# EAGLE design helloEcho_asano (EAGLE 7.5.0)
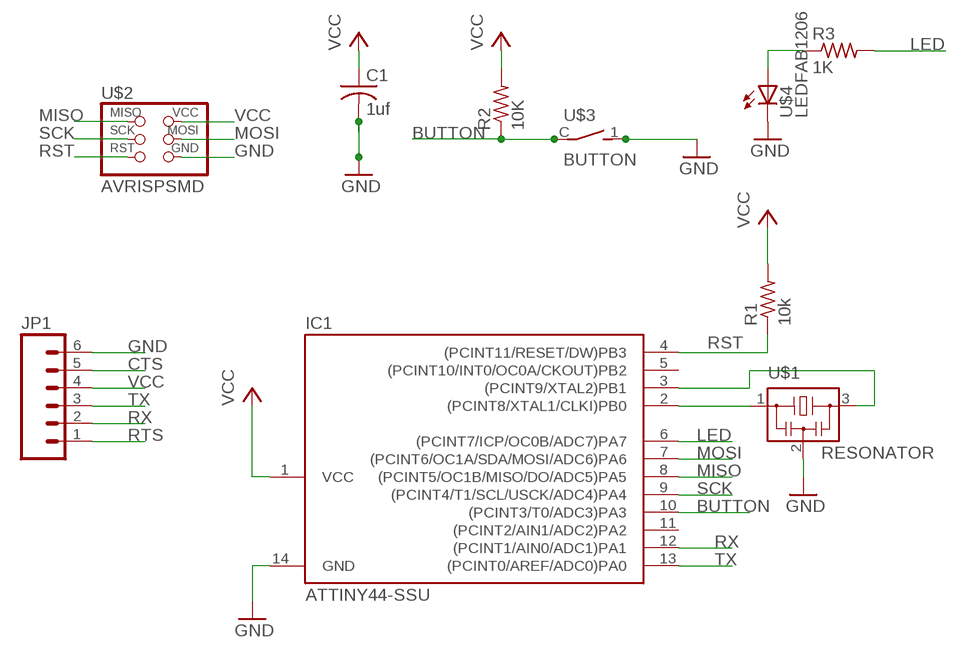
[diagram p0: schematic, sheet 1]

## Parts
C1  1uf  C-USC1206  [C1206]
IC1  ATTINY44-SSU  [SOIC14]
JP1  M06SMD  [1X06-SMD]
R1  10k  R-US_R1206  [R1206]
R2  10K  RES-US1206FAB  [R1206FAB]
R3  1K  RES-US1206FAB  [R1206FAB]
U$1  RESONATOR  [EFOBM]
U$2  AVRISPSMD  [2X03SMD]
U$3  BUTTON  [BUT-NPS]
U$4  LEDFAB1206  [LED1206FAB]

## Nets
BUTTON: IC1.10((PCINT3/T0/ADC3)PA3) R2.1 U$3.C
CTS: JP1.5
GND: C1.2 IC1.14(GND) JP1.6 U$1.2 U$2.6(GND) U$3.1 U$4.2(C)
LED: IC1.6((PCINT7/ICP/OC0B/ADC7)PA7) R3.2
MISO: IC1.8((PCINT5/OC1B/MISO/DO/ADC5)PA5) U$2.1(MISO)
MOSI: IC1.7((PCINT6/OC1A/SDA/MOSI/ADC6)PA6) U$2.4(MOSI)
N$1: IC1.2((PCINT8/XTAL1/CLKI)PB0) U$1.1
N$2: IC1.3((PCINT9/XTAL2)PB1) U$1.3
N$3: R3.1 U$4.1(A)
RST: IC1.4((PCINT11/RESET/DW)PB3) R1.1 U$2.5(RST)
RTS: JP1.1
RX: IC1.12((PCINT1/AIN0/ADC1)PA1) JP1.2
SCK: IC1.9((PCINT4/T1/SCL/USCK/ADC4)PA4) U$2.3(SCK)
TX: IC1.13((PCINT0/AREF/ADC0)PA0) JP1.3
VCC: C1.1 IC1.1(VCC) JP1.4 R1.2 R2.2 U$2.2(VCC)
Unconnected: IC1.5((PCINT10/INT0/OC0A/CKOUT)PB2) IC1.11((PCINT2/AIN1/ADC2)PA2)

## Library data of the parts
C1 = rcl:C-US: CAPACITOR, American symbol
IC1 = fab:ATTINY44
JP1 = SparkFun:M06: Header 6 Standard 6-pin 0.1" header. Use with straight break away headers (SKU : PRT-00116), right angle break away headers (PRT-00553), swiss pins (PRT-00743), machine pins (PRT-00117), and female headers (PRT-00115). Molex polarized connector foot print use with SKU : PRT-08094 with associated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
R1 = resistor:R-US_: RESISTOR, American symbol
R2 R3 = HelloKamakura:RES-US: Resistor (US Symbol)
U$1 = fab:RESONATOR
U$2 = fab:AVRISP
U$3 = HelloKamakura:BUTTON: Distribute : Akizuki Densi
U$4 = HelloKamakura:LED: LED

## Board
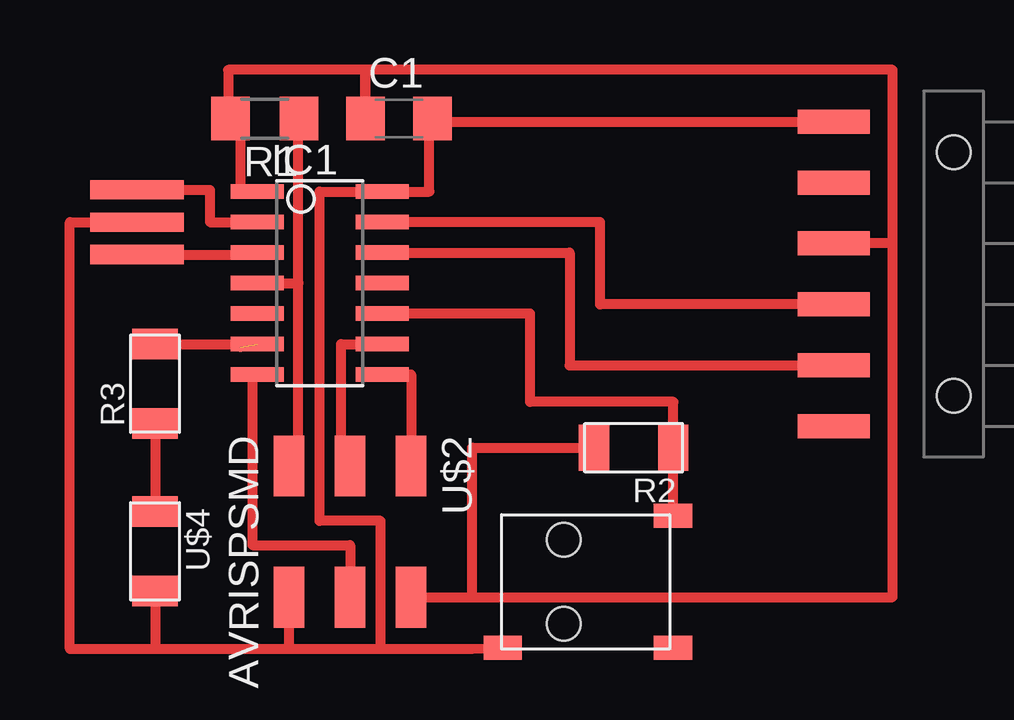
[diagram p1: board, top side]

No outline drawn. Coordinates in mm, seen from the top.
Copper layers 1: Top 0.035mm
Design rules "ERP-1sided-10mil-16mill": minimum track width 10mil, minimum drill 24mil, track to track 16mil, track to pad 16mil, pad to pad 16mil, via to via 16mil, smd to smd 0mil, copper to edge 16mil, drill to drill 36mil, minimum pad ring 10mil, minimum via ring 8mil, stop-mask expansion 4mil, vias tented up to drill 0mil, thermal gap 10mil

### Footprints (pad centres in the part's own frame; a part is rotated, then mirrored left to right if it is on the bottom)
C1206 = smd 1.6 x 1.8: 1 -1.4,0; 2 1.4,0
SOIC14 = smd 0.61 x 2.21: 1 -3.81,-2.603; 2 -2.54,-2.603; 3 -1.27,-2.603; 4 0,-2.603; 5 1.27,-2.603; 6 2.54,-2.603; 7 3.81,-2.603; 8 3.81,2.603; 9 2.54,2.603; 10 1.27,2.603; 11 0,2.603; 12 -1.27,2.603; 13 -2.54,2.603; 14 -3.81,2.603
1X06-SMD = smd 1 x 3: 1 -6.35,5; 2 -3.81,5; 3 -1.27,5; 4 1.27,5; 5 3.81,5; 6 6.35,5 | hole 1.4: -5.08,0; 5.08,0
R1206 = smd 1.6 x 1.803: 1 -1.422,0; 2 1.422,0
R1206FAB = smd 1.27 x 1.905: 1 -1.651,0; 2 1.651,0
EFOBM = smd 0.8 x 3.9: 1 -1.35,0; 2 0,0; 3 1.35,0
2X03SMD = smd 2.54 x 1.27: 1 -2.54,2.54; 2 2.92,2.54; 3 -2.54,0; 4 2.92,0; 5 -2.54,-2.54; 6 2.92,-2.54
BUT-NPS = smd 1 x 1.6: 1 2.75,-3.55; C -2.75,3.55; P$1 2.75,3.55 | hole 1.4: -1.75,-1; 1.75,-1
LED1206FAB = smd 1.27 x 1.905: 1 -1.651,0; 2 1.651,0

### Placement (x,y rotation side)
C1  29.72,40.51 0 top
IC1  26.42,33.66 270 top
JP1  52.83,34.04 90 top
R1  24.13,40.51 180 top
R2  39.5,26.8 180 top
R3  19.56,29.46 90 top
U$1  18.8,36.2 270 top
U$2  27.69,23.5 270 top
U$3  37.59,21.21 270 top
U$4  19.56,22.48 270 top

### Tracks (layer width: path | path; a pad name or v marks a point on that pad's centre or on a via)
BUTTON
  Top 0.406: U$3.C R2.1 41.15,28.7 35.18,28.7 35.18,32.38 IC1.10
GND
  Top 0.406: 28.96,18.41 28.96,23.75 26.42,23.75 26.42,37.47 IC1.14 30.99,37.47 30.99,40.51 C1.2 31.12,40.39 JP1.6 47.83,40.64 | 25.15,18.41 28.96,18.41 | U$1.2 16,36.2 16,18.41 19.56,18.41 | U$2.6 25.15,18.41 | 19.56,18.41 25.15,18.41 | 28.96,18.41 32.77,18.41 U$3.1 | U$4.2 19.56,18.41
LED  (1 unrouted)
  Top 0.406: R3.2 23.11,31.11 23.11,30.99
MISO
  Top 0.406: IC1.8 30.23,29.84 U$2.1
MOSI
  Top 0.406: IC1.7 23.62,29.84 23.62,22.73 27.69,22.73 U$2.4
N$1
  Top 0.406: U$1.1 21.84,37.55 21.84,36.2 IC1.2
N$2
  Top 0.406: U$1.3 23.81,34.84 IC1.3
N$3
  Top 0.406: R3.1 U$4.1
RST
  Top 0.406: R1.1 25.53,40.51 25.53,33.66 | IC1.4 25.53,33.66 | U$2.5 25.53,26.04 25.53,33.66
RX
  Top 0.406: IC1.12 36.83,34.92 36.83,30.23 JP1.2
SCK
  Top 0.406: U$2.3 27.3,26.04 27.3,31.11 IC1.9
TX
  Top 0.406: JP1.3 38.1,32.77 38.1,36.2 IC1.13
VCC
  Top 0.254: 50.29,21.72 50.29,21.82
  Top 0.406: 50.29,35.31 JP1.4 | 50.29,35.31 50.29,21.72 50.29,20.57 U$2.2 32.77,20.57 32.77,26.8 R2.2 | IC1.1 23.11,37.47 23.11,40.51 R1.2 22.61,40.51 22.61,42.55 28.32,42.55 C1.1 28.32,42.55 50.29,42.55 50.29,35.31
